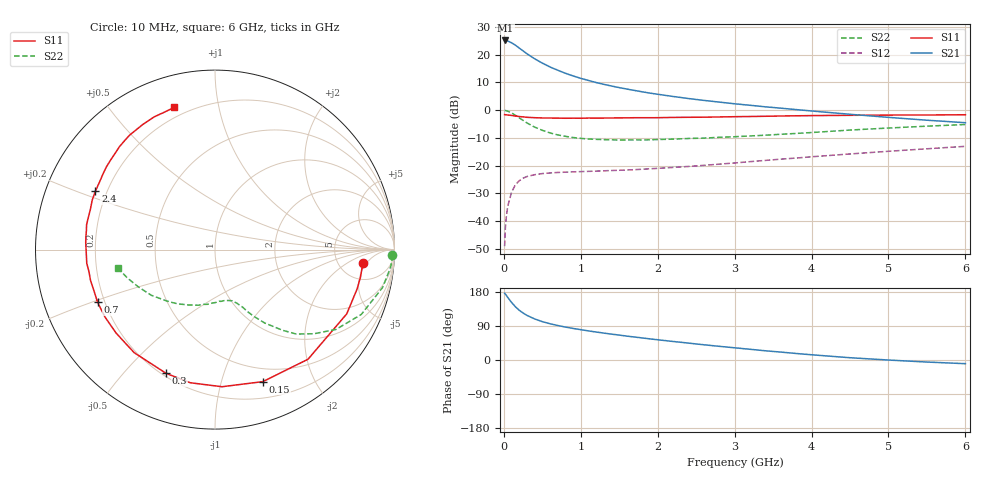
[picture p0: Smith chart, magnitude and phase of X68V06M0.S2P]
! SIEMENS Small Signal Semiconductors
! BFP193W
! Si NPN RF Bipolar Junction Transistor in SOT343
! VCE = 8 V  IC = 6 mA
! Common Emitter S-Parameters:  April 1994
# GHz  S  MA  R  50
!  f  S11  S21  S12  S22
! GHz  MAG  ANG  MAG  ANG  MAG  ANG  MAG  ANG
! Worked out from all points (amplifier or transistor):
!   40 points, 10 MHz to 6 GHz, reference 50 ohm
!   highest |S21| = 25.1 dB at 20 MHz (marker M1)
!   |S21| within 3 dB of that: start of sweep to 212.8 MHz
!   unconditionally stable (mu >= 1): 1.655 GHz to 4.54 GHz
!   at 200 MHz: K = 0.16, MSG = 24.0 dB, |S12| = -25.5 dB
!   at 1.5 GHz: K = 0.94, MSG = 14.9 dB, |S12| = -21.7 dB
!   at 6 GHz: K = 0.91, MSG = 4.3 dB, |S12| = -13.1 dB
!   lowest NFmin = 1.20 dB at 450 MHz
!   S11 on the Smith chart (normalised r, x): 10 MHz: 8.61, -4.09; 150 MHz: 0.36, -1.36; 300 MHz: 0.22, -0.66; 700 MHz: 0.17, -0.21; 2.4 GHz: 0.16, +0.23; 6 GHz: 0.15, +0.74
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0.01  0.8272 -5.2  18.04 176.0  0.0035 89.1  0.9887 -1.8
0.02  0.8251 -10.5  18.07 174.0  0.0076 82.0  0.9844 -5.3
0.05  0.8167 -26.0  17.68 165.4  0.0182 76.9  0.9569 -12.8
0.1  0.8011 -49.7  16.42 152.1  0.0329 65.3  0.8916 -23.9
0.15  0.7824 -70.1  14.85 140.5  0.0448 55.5  0.8077 -33.4
0.2  0.765 -87.1  13.18 131.3  0.053 48.4  0.7237 -40.4
0.25  0.7545 -100.5  11.72 124.0  0.059 42.8  0.6527 -46.1
0.3  0.7412 -111.6  10.4 117.8  0.0633 38.4  0.5873 -50.0
0.4  0.7298 -128.1  8.446 108.4  0.0682 32.5  0.4939 -55.9
0.5  0.7211 -139.8  7.044 101.2  0.0715 29.0  0.4316 -59.7
0.6  0.7189 -148.5  6.002 95.7  0.0733 26.9  0.3876 -62.5
0.7  0.7171 -155.8  5.252 91.1  0.0749 25.7  0.3567 -64.3
0.9  0.7145 -166.1  4.142 83.3  0.0768 24.7  0.32 -68.1
1.1  0.7186 -173.9  3.43 76.8  0.0784 25.1  0.3003 -71.6
1.3  0.7183 179.7  2.914 71.0  0.0802 26.0  0.2931 -75.3
1.6  0.7244 171.4  2.397 63.0  0.0831 28.6  0.2891 -80.8
2.2  0.7376 158.0  1.763 48.9  0.0923 34.0  0.299 -93.4
2.4  0.7417 153.9  1.618 44.6  0.0961 35.6  0.3074 -97.5
3.2  0.7663 139.4  1.222 28.3  0.1174 40.4  0.3414 -115.3
4.5  0.8049 120.0  0.841 6.0  0.1616 40.7  0.4364 -144.3
5.5  0.8157 110.4  0.657 -5.4  0.2003 37.3  0.513 -162.0
6  0.8244 105.9  0.592 -9.7  0.2217 35.3  0.5494 -169.0
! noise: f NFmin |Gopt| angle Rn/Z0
0.45  1.2  0.25  114  0.13
0.9  1.25  0.37  150  0.12
1.8  2  0.55  -158  0.12
